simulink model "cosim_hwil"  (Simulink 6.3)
settings: Solver=ode45  StartTime=0.0  StopTime=1000  RelTol=1e-3
undefined symbols (not defined in the file or in its folder): cosim_xrc4_top, netlist_xrc4
libraries: adcosim_example_lib x1

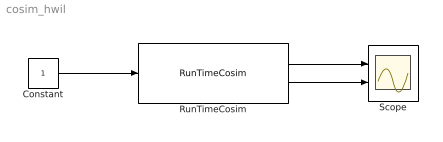
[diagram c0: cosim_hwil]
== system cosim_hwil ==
  Constant : Constant
  RunTimeCosim : adcosim_example_lib/RunTimeCosim  index=0  bitstream=netlist_xrc4/cosim_xrc4_top.bit  freq=120  single_step=on  shared=None
  Scope : Scope  NumInputPorts=2
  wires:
  Constant/1 -> RunTimeCosim/1
  RunTimeCosim/1 -> Scope/1
  RunTimeCosim/2 -> Scope/2
